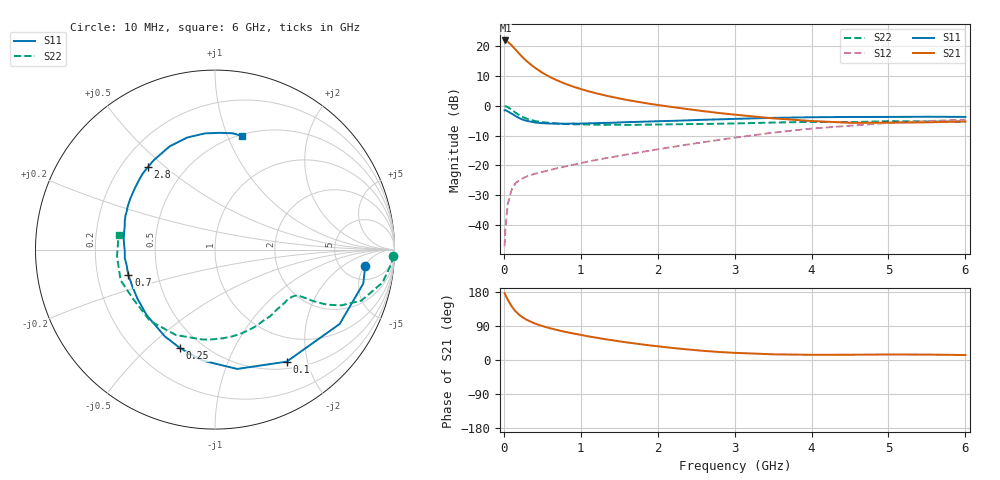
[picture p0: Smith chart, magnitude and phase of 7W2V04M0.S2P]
! Infineon Technologies  Discrete & RF Semiconductors
! BFS17W
! Si NPN RF Bipolar Junction Transistor in SOT323
! VCE = 2 V  IC = 4 mA
! Common Emitter S-Parameters:  August  1999
# GHz  S  MA  R  50
!  f  S11  S21  S12  S22
! GHz  MAG  ANG  MAG  ANG  MAG  ANG  MAG  ANG
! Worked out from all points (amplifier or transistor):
!   36 points, 10 MHz to 6 GHz, reference 50 ohm
!   highest |S21| = 22.0 dB at 20 MHz (marker M1)
!   |S21| within 3 dB of that: start of sweep to 149.4 MHz
!   unconditionally stable (mu >= 1): 587.3 MHz to end of sweep
!   at 250 MHz: K = 0.54, MSG = 20.2 dB, |S12| = -24.3 dB
!   at 1.4 GHz: K = 1.30, MAG = 6.9 dB, |S12| = -17.3 dB
!   at 6 GHz: K = 1.10, MAG = -2.3 dB, |S12| = -4.6 dB
!   S11 on the Smith chart (normalised r, x): 10 MHz: 8.36, -5.22; 100 MHz: 0.60, -1.66; 250 MHz: 0.38, -0.64; 700 MHz: 0.34, -0.13; 2.8 GHz: 0.31, +0.44; 6 GHz: 0.51, +1.13
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0.01  0.8419 -6.2  12.51 176.4  0.0044 83.1  0.9945 -1.9
0.02  0.8476 -12.9  12.52 171.6  0.0085 84.9  0.985 -4.7
0.05  0.8089 -30.8  11.91 159.2  0.022 75.6  0.9516 -11.1
0.1  0.741 -57.4  10.43 142.3  0.0387 61.9  0.8637 -19.2
0.15  0.6763 -79.5  8.844 128.9  0.0499 53.8  0.7693 -23.8
0.2  0.6223 -96.2  7.515 119.2  0.0564 49.9  0.6985 -26.1
0.25  0.5828 -109.4  6.417 111.7  0.0612 45.7  0.6443 -27.2
0.3  0.5583 -120.1  5.577 105.8  0.0652 44.8  0.6082 -27.8
0.4  0.5273 -136.4  4.389 96.5  0.0719 44.4  0.5578 -28.4
0.5  0.5111 -147.9  3.599 89.7  0.0777 45.2  0.5325 -28.9
0.6  0.5038 -156.5  3.043 83.8  0.0836 46.9  0.5151 -29.9
0.7  0.5031 -163.7  2.649 78.8  0.09 48.3  0.5037 -31.4
0.9  0.5046 -174.7  2.104 70.1  0.1021 51.4  0.4894 -35.2
1.1  0.5081 176.4  1.757 62.3  0.1164 53.9  0.4843 -39.8
1.3  0.5159 168.8  1.514 55.5  0.1304 55.9  0.4793 -45.2
1.6  0.5332 159.5  1.255 46.4  0.1524 58.2  0.479 -53.5
2.2  0.5599 143.8  0.95 31.6  0.2048 60.8  0.4895 -71.9
2.8  0.5928 129.2  0.757 21.1  0.2678 60.0  0.5 -91.5
3.5  0.6284 113.7  0.616 15.0  0.3546 55.5  0.5234 -114.5
4.5  0.6498 95.0  0.519 13.9  0.4632 43.8  0.5318 -148.2
5.5  0.6554 81.6  0.528 14.3  0.5531 31.8  0.5472 -176.2
6  0.6517 76.6  0.547 13.1  0.5877 26.0  0.5429 171.4
